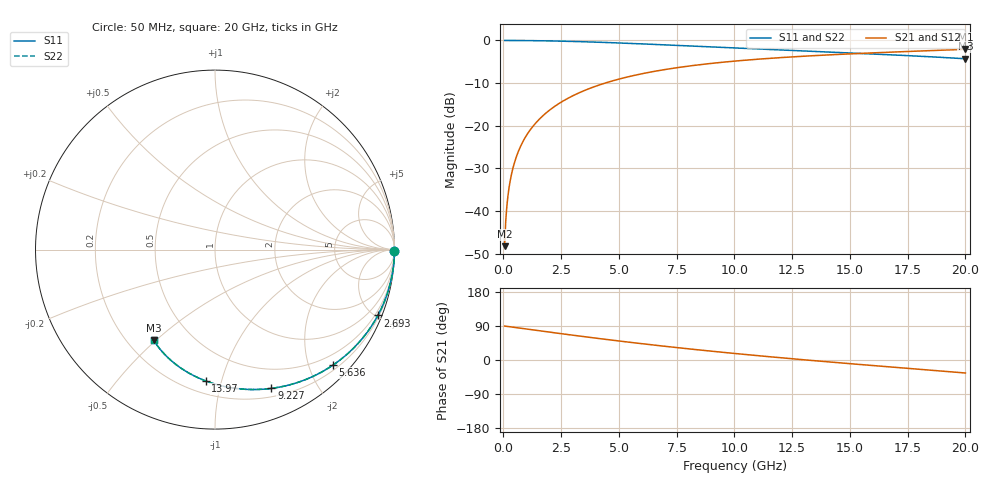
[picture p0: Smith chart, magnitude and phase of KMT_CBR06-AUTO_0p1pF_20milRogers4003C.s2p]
! Data measured by Modelithics Inc. support@modelithics.com 813-866-6335
! KEMET CBR06-AUTO 0.1pF, Pad Width= 0.851mm, Pad Length= 0.64mm, Pad Gap= 0.62mm, 20mil Rogers 4003C substrate Data, January 2022
# hz S ma R 50
! 2 Port Network Data from SP1.SP block
! freq  magS11  angS11  magS21  angS21  magS12  angS12  magS22  angS22
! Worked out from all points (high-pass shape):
!   401 points, 50 MHz to 20 GHz, reference 50 ohm
!   highest |S21| = -2.08 dB at 20 GHz (marker M1); lowest = -48.2 dB at 50 MHz (marker M2)
!   |S21| within 3 dB of the highest: 9.54 GHz to end of sweep
!   lowest |S11| = -4.3 dB at 20 GHz (marker M3), VSWR 4.13, Z = 15.3 - j24.7 ohm
!   |S11| at or under -10 dB: nowhere
!   |S22| runs from -4.3 to 0.0 dB; largest |S21 - S12| = 0
!   S11 on the Smith chart (normalised r, x): 50 MHz: open; 2.693 GHz: 0.29, -5.12; 5.636 GHz: 0.29, -2.43; 9.227 GHz: 0.28, -1.45; 13.97 GHz: 0.28, -0.89; 20 GHz: 0.31, -0.49
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5e7  1 -0.4  0.003889 89.6  0.003889 89.6  1 -0.4
9.9875e7  1 -0.8  0.007768 89.2  0.007768 89.2  1 -0.8
1.99625e8  0.9999 -1.7  0.01552 88.3  0.01552 88.3  0.9999 -1.7
2.495e8  0.9998 -2.1  0.0194 87.9  0.0194 87.9  0.9998 -2.1
2.99375e8  0.9997 -2.5  0.02328 87.5  0.02328 87.5  0.9997 -2.5
3.99125e8  0.9995 -3.3  0.03102 86.7  0.03102 86.7  0.9995 -3.3
4.98875e8  0.9992 -4.1  0.03876 85.9  0.03876 85.9  0.9992 -4.1
7.4825e8  0.9983 -6.2  0.05806 83.8  0.05806 83.8  0.9983 -6.2
1.097375e9  0.9963 -9.1  0.08491 80.9  0.08491 80.9  0.9963 -9.1
1.496375e9  0.9932 -12.4  0.1153 77.6  0.1153 77.6  0.9932 -12.4
2.045e9  0.9875 -16.8  0.1562 73.1  0.1562 73.1  0.9875 -16.8
2.693375e9  0.9788 -22.0  0.2032 67.9  0.2032 67.9  0.9788 -22.0
3.391625e9  0.9673 -27.5  0.2515 62.4  0.2515 62.4  0.9673 -27.5
4.439e9  0.9469 -35.5  0.3191 54.3  0.3191 54.3  0.9469 -35.5
5.636e9  0.9203 -44.3  0.3883 45.6  0.3883 45.6  0.9203 -44.3
6.73325e9  0.8942 -51.9  0.4441 37.9  0.4441 37.9  0.8942 -51.9
9.227e9  0.8347 -67.9  0.5466 21.9  0.5466 21.9  0.8347 -67.9
1.0025e10  0.8163 -72.6  0.5733 17.1  0.5733 17.1  0.8163 -72.6
1.336662e10  0.7453 -91.0  0.6621 -1.3  0.6621 -1.3  0.7453 -91.0
1.396512e10  0.7334 -94.1  0.6752 -4.4  0.6752 -4.4  0.7334 -94.1
1.670825e10  0.6799 -107.8  0.7286 -18.2  0.7286 -18.2  0.6799 -107.8
2e10  0.6103 -123.9  0.7874 -34.3  0.7874 -34.3  0.6103 -123.9
